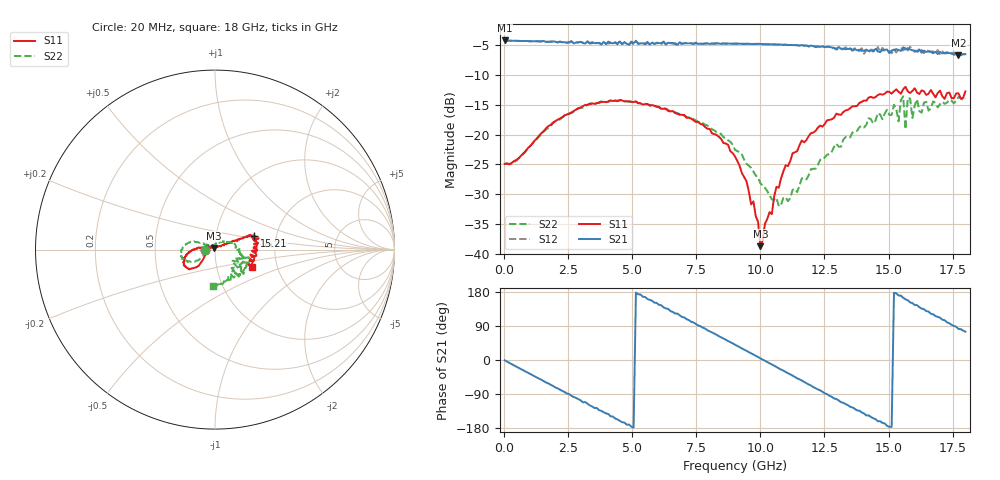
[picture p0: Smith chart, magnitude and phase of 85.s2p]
!Agilent Technologies,N5230A,US43500223,A.07.50.48
!Agilent N5230A: A.07.50.48
!Date: Monday, January 11, 2016 19:58:53
!Correction: S11(Full 2 Port(1,2))
!S21(Full 2 Port(1,2))
!S12(Full 2 Port(1,2))
!S22(Full 2 Port(1,2))
!S2P File: Measurements: S11, S21, S12, S22:
# Hz S  dB  R 50
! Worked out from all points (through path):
!   201 points, 20 MHz to 18 GHz, reference 50 ohm
!   highest |S21| = -4.21 dB at 20 MHz (marker M1); lowest = -6.7 dB at 17.73 GHz (marker M2)
!   group delay of S21, straight-line fit = 99.5 ps
!   lowest |S11| = -38.7 dB at 9.999 GHz (marker M3), VSWR 1.02, Z = 49.3 + j0.936 ohm
!   |S11| at or under -10 dB: start of sweep to end of sweep
!   |S22| runs from -32.0 to -13.6 dB; largest |S21 - S12| = 0.051
!   S11 on the Smith chart (normalised r, x): 20 MHz: 0.89, -0.00; 15.21 GHz: 1.54, +0.24; 18 GHz: 1.48, -0.31
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2e7  -24.95 -179.8  -4.21 -0.8  -4.22 -0.8  -24.91 -179.0
1.5483e9  -19.41 -137.0  -4.30 -56.0  -4.33 -55.9  -19.49 -147.4
3.0766e9  -15.26 -142.1  -4.65 -111.7  -4.54 -110.5  -15.51 -157.3
4.515e9  -14.22 -153.8  -4.39 -160.4  -4.25 -159.4  -14.25 -172.5
6.0433e9  -15.45 -167.4  -4.66 145.5  -4.64 144.9  -15.37 171.6
7.4817e9  -17.90 -179.0  -4.57 95.1  -4.72 95.0  -17.62 161.6
9.01e9  -23.68 173.7  -4.77 40.6  -4.71 40.6  -22.57 154.1
9.7292e9  -31.23 154.7  -4.80 14.6  -4.79 14.7  -26.22 147.1
9.9989e9  -38.74 124.9  -4.81 4.3  -4.81 4.6  -28.17 142.5
1.07181e10  -28.95 28.4  -4.91 -21.5  -4.91 -21.6  -32.03 113.2
1.20666e10  -19.67 23.9  -5.18 -71.6  -5.17 -71.1  -25.76 55.2
1.33252e10  -15.95 22.5  -5.69 -116.4  -5.36 -116.0  -20.44 24.6
1.50333e10  -12.86 18.4  -6.34 -176.2  -6.00 -177.1  -16.71 -20.9
1.52131e10  -12.73 18.8  -5.76 177.5  -5.64 179.1  -15.02 -16.7
1.53929e10  -12.83 15.7  -5.80 170.1  -5.66 174.9  -17.80 -22.7
1.55727e10  -12.40 14.7  -5.36 164.3  -5.89 168.6  -13.59 -40.4
1.56626e10  -11.99 14.5  -5.74 160.0  -5.30 161.4  -19.12 -33.7
1.57525e10  -12.76 13.3  -5.50 157.8  -5.89 155.7  -13.84 -21.9
1.59323e10  -12.68 11.6  -5.86 150.2  -5.69 148.1  -17.22 -47.9
1.61121e10  -12.95 8.7  -6.07 144.9  -5.91 142.0  -14.08 -45.0
1.77303e10  -13.09 -24.8  -6.70 82.0  -6.32 84.2  -13.72 -88.9
1.8e10  -12.77 -25.6  -6.51 74.8  -6.53 73.5  -13.92 -92.9
